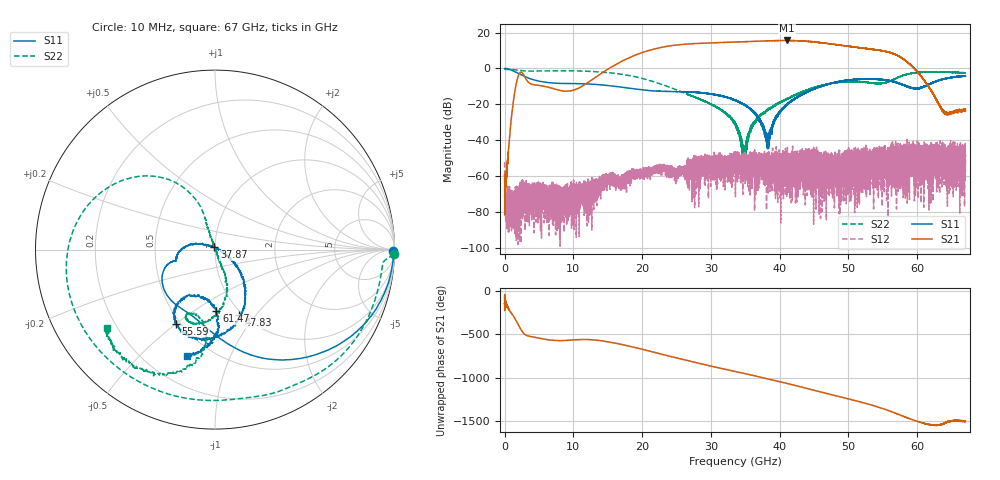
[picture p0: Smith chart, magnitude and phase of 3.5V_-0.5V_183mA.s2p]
! MARKI MICROWAVE INC.
! Date:  10/21/2020
! Model Number:  AMM-7210CH
! Description:  2-port Small Signal S-parameter data for AMM-7210CH
! Frequency Range:  10 MHz to 67 GHz
! Port Configuration:  PORT 1: Input
!  PORT 2: Output
! Bias Condition: Vd = +3.5V, Vg = -0.5V
! AMM-7210CH s2p files are only valid for small signal conditions (below -10 dBm input power)
# Hz S  dB  R 50
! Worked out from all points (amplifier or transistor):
!   20001 points, 10 MHz to 67 GHz, reference 50 ohm
!   highest |S21| = 15.6 dB at 41.06 GHz (marker M1)
!   |S21| within 3 dB of that: 24.1 GHz to 49.48 GHz (25.38 GHz wide, 69 % of centre)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
!   unconditionally stable (mu >= 1): start of sweep to end of sweep
!   at 11.17 GHz: K = 1185.84, MAG = -4.2 dB, |S12| = -69.3 dB
!   at 33.51 GHz: K = 41.42, MAG = 14.8 dB, |S12| = -53.2 dB
!   at 67 GHz: K = 896.39, MAG = -18.2 dB, |S12| = -52.4 dB
!   S11 on the Smith chart (normalised r, x): 10 MHz: open; 37.87 GHz: 0.99, +0.03; 47.83 GHz: 0.96, -0.83; 55.59 GHz: 0.47, -0.50; 61.47 GHz: 0.80, -0.62; 67 GHz: 0.38, -0.70
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1e7  -0.06 -0.6  -59.62 -142.0  -52.33 162.5  -0.02 -1.5
2.227369e9  -3.23 -62.7  -2.52 -60.8  -67.02 9.2  -1.19 -61.7
1.117723e10  -8.57 -132.8  -10.21 162.1  -67.56 -176.9  -1.50 -168.6
1.702546e10  -10.50 -159.7  3.90 105.2  -61.75 123.4  -3.30 149.0
1.991608e10  -11.95 -164.2  8.67 51.7  -60.63 118.8  -5.49 129.8
2.234112e10  -12.76 -163.8  11.33 2.9  -55.20 114.1  -8.28 116.8
2.462548e10  -12.97 -165.2  12.83 -43.3  -59.09 79.9  -11.42 109.3
2.764338e10  -13.32 -170.9  13.84 -101.3  -56.97 77.2  -16.06 108.1
3.081535e10  -14.91 178.1  14.33 -158.4  -55.07 57.0  -21.79 109.1
3.3505e10  -17.86 167.3  14.69 154.6  -53.20 24.0  -30.25 103.7
3.787275e10  -37.06 106.8  15.30 77.1  -50.13 -13.0  -24.29 -64.9
4.106147e10  -20.23 -29.7  15.58 16.8  -58.52 -147.8  -17.02 -68.7
4.274962e10  -15.84 -39.5  15.39 -17.0  -50.44 -152.6  -14.00 -71.7
4.467223e10  -11.91 -50.2  14.93 -55.8  -56.78 -145.0  -11.16 -77.6
4.783081e10  -8.16 -69.6  13.44 -118.9  -54.78 -66.7  -8.14 -93.9
5.128415e10  -6.12 -92.3  11.72 172.3  -53.71 139.0  -7.34 -111.4
5.368909e10  -5.90 -107.0  10.53 120.0  -57.07 -157.1  -8.31 -111.9
5.559495e10  -6.62 -117.9  9.28 70.5  -50.20 168.5  -7.78 -100.1
5.583612e10  -6.78 -118.9  9.04 63.8  -57.65 35.2  -7.37 -98.3
5.86028e10  -10.38 -120.5  3.34 -20.5  -47.53 -99.7  -3.16 -104.6
6.147332e10  -9.28 -88.7  -9.20 -92.1  -59.00 122.4  -1.94 -123.3
6.7e10  -4.41 -104.8  -23.76 -57.1  -52.38 22.8  -2.51 -144.5
